(* Logix 5000 AddOnInstructionDefinition export AMP_Tuning_Params_StepSERVO; software revision 20.04 *)

ADD_ON_INSTRUCTION AMP_Tuning_Params_StepSERVO   (* revision 1.0 *)
// Applied Motion - Tuning Parameters StepSERVO AOI
// Help:
// The Tuning Parameters for StepSERVO AOI accepts all the required parameters for SCL commands VP, VI, KK, KC, KP, KD and KE, and then scales and issues these to the drive, one at a time.
VAR_IN_OUT
   MSG_Write : SINT[8]; {required}   // Message Write data tag
        [0]   // Message Reserved = 0
        [1]   // Message Type (16#01 or 16#02)
        [2]   // Type 1: Register Type 2: Opcode
        [3]   // Type 1: Opcode Type 2: Operand
        [4]   // Type 1: Parameter 1 Type 2: data MSB
        [5]   // Type 1: Parameter 2 Type 2: data LSB
        [6]   // Type 1: Parameter 3 Type 2: not used
        [7]   // Type 1: Parameter 4 Type 2: not used
   SendMsg : MESSAGE; {required}   // Message tag
   MSG_Response : SINT[8]; {required}   // Message Response data tag
        [0]   // Command Word
        [1]   // Jog Speed (0.25 rev/min)
        [2]   // Jog Acceleration (10 rev/s/s)
        [3]   // Jog Deceleration (10 rev/s/s)
        [4]   // Point-to-Point Velocity (0.25 rev/min)
        [5]   // Point-to-Point Acceleration (10 rev/s/s)
        [6]   // Point-to-Point Deceleration (10 rev/s/s)
        [7]   // Point-to-Point Distance (Motor steps)
        [9]   // (2x ASCII Letters in 16 lower word)
        [10]   // Data/Register 1
        [11]   // Data/Register 2
END_VAR
VAR_INPUT
   Configure : BOOL; {required}   // Start the Configuration
   VP : INT; {required}   // Velocity Mode Proportional Constant
   VI : INT; {required}   // Velocity Integrator Constant
   KP : INT; {required}   // Proportional Global Gain Value
   KK : INT; {required}   // Inertia Feedforward Gain
   KE : INT; {required}   // Differential Filter Gain Value
   KD : INT; {required}   // Damping Gain Value
   KC : INT; {required}   // Overall Servo Filter value
END_VAR
VAR_OUTPUT
   Sent : BOOL; {access Read Only, visible}   // All parameter settings have been sent to drive
   In_Progress : BOOL; {access Read Only, visible}   // The setting of parameters is in progress
   Done : BOOL; {access Read Only, visible}   // Parameters set without errors
   Error : BOOL; {access Read Only, visible}   // Configuration failed to complete - drive not ready or faulted
   State : DINT := 34; {access Read Only}   // Internal state of progress
END_VAR
VAR
   Loc_Start_ONS : BOOL; {access None}
   MSG_Active : BOOL;
END_VAR

ROUTINE Logic   (* ladder *)
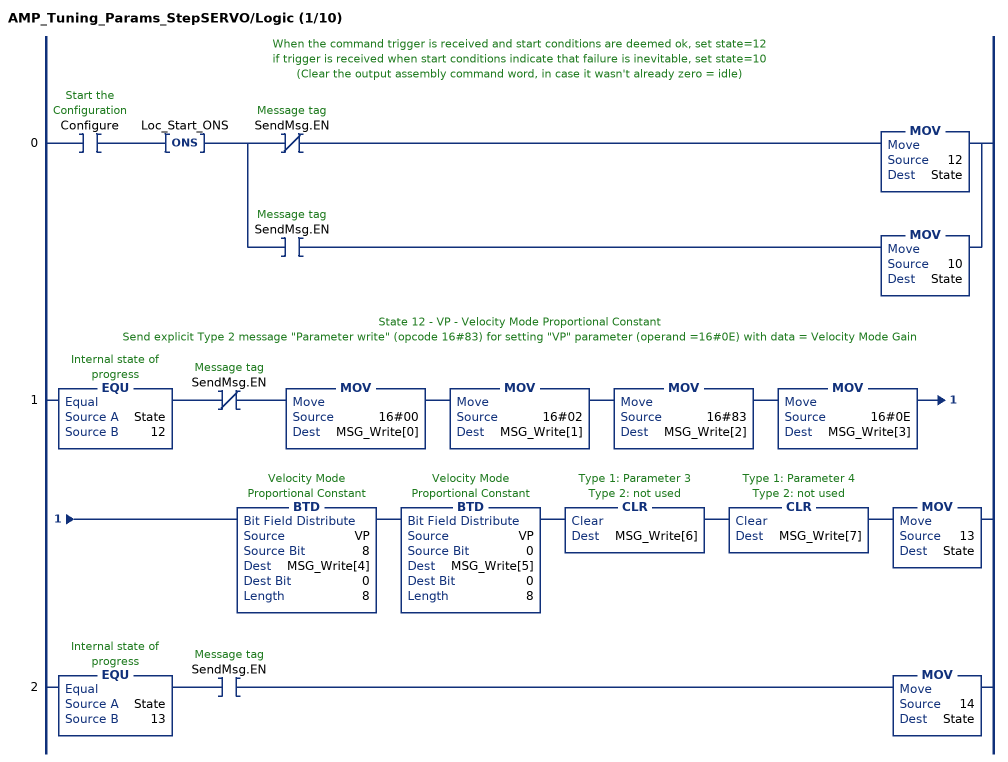
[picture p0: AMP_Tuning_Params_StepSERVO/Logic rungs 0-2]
   // When the command trigger is received and start conditions are deemed ok, set state=12
   // if trigger is received when start conditions indicate that failure is inevitable, set state=10
   // (Clear the output assembly command word, in case it wasn't already zero = idle)
   0: XIC(Configure)ONS(Loc_Start_ONS)[XIO(SendMsg.EN) MOV(12,State) ,XIC(SendMsg.EN) MOV(10,State) ];
   // State 12 - VP - Velocity Mode Proportional Constant
   // Send explicit Type 2 message "Parameter write" (opcode 16#83) for setting "VP" parameter (operand =16#0E) with data = Velocity Mode Gain
   1: EQU(State,12)XIO(SendMsg.EN)MOV(16#00,MSG_Write[0])MOV(16#02,MSG_Write[1])MOV(16#83,MSG_Write[2])MOV(16#0E,MSG_Write[3])BTD(VP,8,MSG_Write[4],0,8)BTD(VP,0,MSG_Write[5],0,8)CLR(MSG_Write[6])CLR(MSG_Write[7])MOV(13,State);
   2: EQU(State,13)XIC(SendMsg.EN)MOV(14,State);
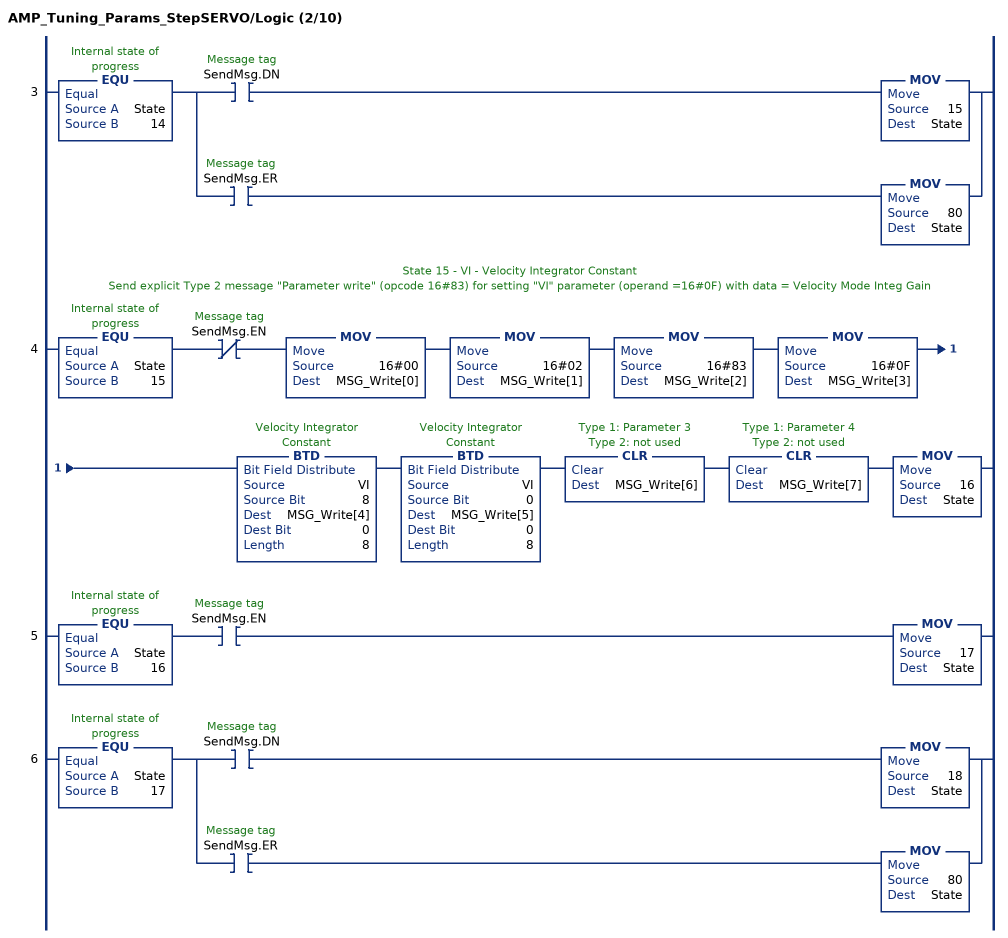
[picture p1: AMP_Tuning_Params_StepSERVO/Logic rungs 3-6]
   3: EQU(State,14)[XIC(SendMsg.DN) MOV(15,State) ,XIC(SendMsg.ER) MOV(80,State) ];
   // State 15 - VI - Velocity Integrator Constant
   // Send explicit Type 2 message "Parameter write" (opcode 16#83) for setting "VI" parameter (operand =16#0F) with data = Velocity Mode Integ Gain
   4: EQU(State,15)XIO(SendMsg.EN)MOV(16#00,MSG_Write[0])MOV(16#02,MSG_Write[1])MOV(16#83,MSG_Write[2])MOV(16#0F,MSG_Write[3])BTD(VI,8,MSG_Write[4],0,8)BTD(VI,0,MSG_Write[5],0,8)CLR(MSG_Write[6])CLR(MSG_Write[7])MOV(16,State);
   5: EQU(State,16)XIC(SendMsg.EN)MOV(17,State);
   6: EQU(State,17)[XIC(SendMsg.DN) MOV(18,State) ,XIC(SendMsg.ER) MOV(80,State) ];
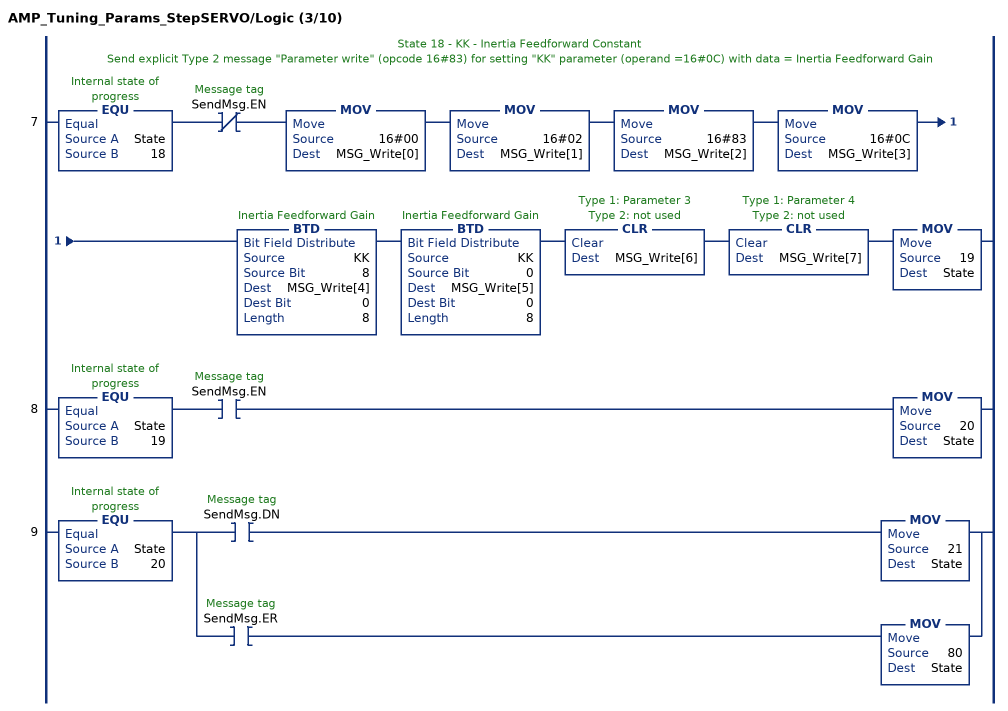
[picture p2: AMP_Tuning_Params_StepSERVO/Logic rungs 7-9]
   // State 18 - KK - Inertia Feedforward Constant
   // Send explicit Type 2 message "Parameter write" (opcode 16#83) for setting "KK" parameter (operand =16#0C) with data = Inertia Feedforward Gain
   7: EQU(State,18)XIO(SendMsg.EN)MOV(16#00,MSG_Write[0])MOV(16#02,MSG_Write[1])MOV(16#83,MSG_Write[2])MOV(16#0C,MSG_Write[3])BTD(KK,8,MSG_Write[4],0,8)BTD(KK,0,MSG_Write[5],0,8)CLR(MSG_Write[6])CLR(MSG_Write[7])MOV(19,State);
   8: EQU(State,19)XIC(SendMsg.EN)MOV(20,State);
   9: EQU(State,20)[XIC(SendMsg.DN) MOV(21,State) ,XIC(SendMsg.ER) MOV(80,State) ];
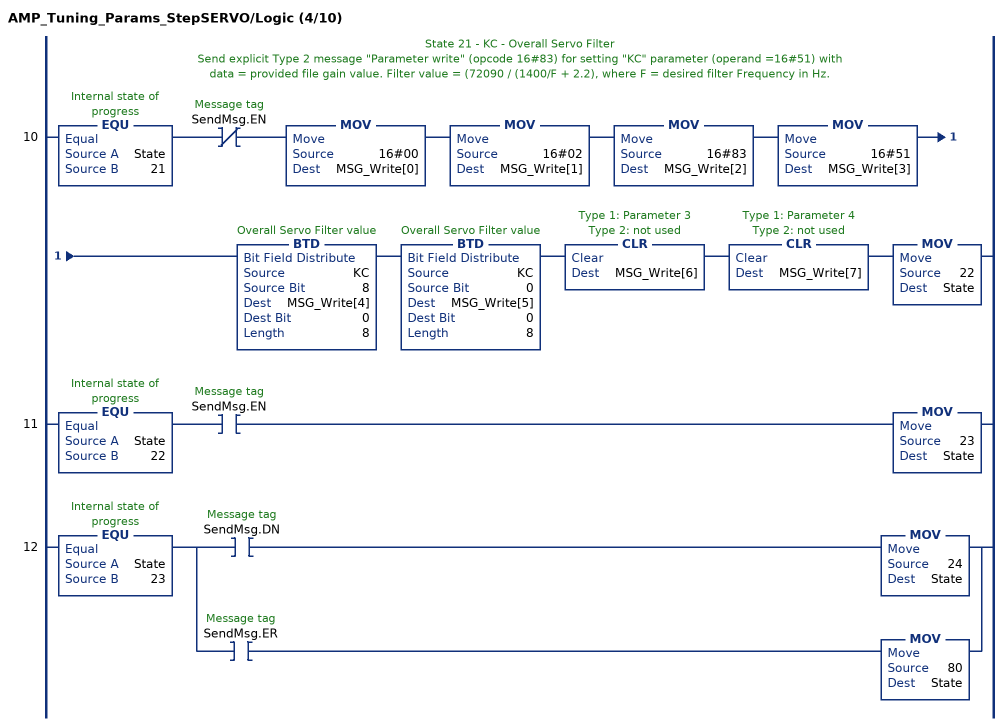
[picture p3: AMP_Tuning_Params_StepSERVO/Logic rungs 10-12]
   // State 21 - KC - Overall Servo Filter
   // Send explicit Type 2 message "Parameter write" (opcode 16#83) for setting "KC" parameter (operand =16#51) with
   // data = provided file gain value. Filter value = (72090 / (1400/F + 2.2), where F = desired filter Frequency in Hz.
   10: EQU(State,21)XIO(SendMsg.EN)MOV(16#00,MSG_Write[0])MOV(16#02,MSG_Write[1])MOV(16#83,MSG_Write[2])MOV(16#51,MSG_Write[3])BTD(KC,8,MSG_Write[4],0,8)BTD(KC,0,MSG_Write[5],0,8)CLR(MSG_Write[6])CLR(MSG_Write[7])MOV(22,State);
   11: EQU(State,22)XIC(SendMsg.EN)MOV(23,State);
   12: EQU(State,23)[XIC(SendMsg.DN) MOV(24,State) ,XIC(SendMsg.ER) MOV(80,State) ];
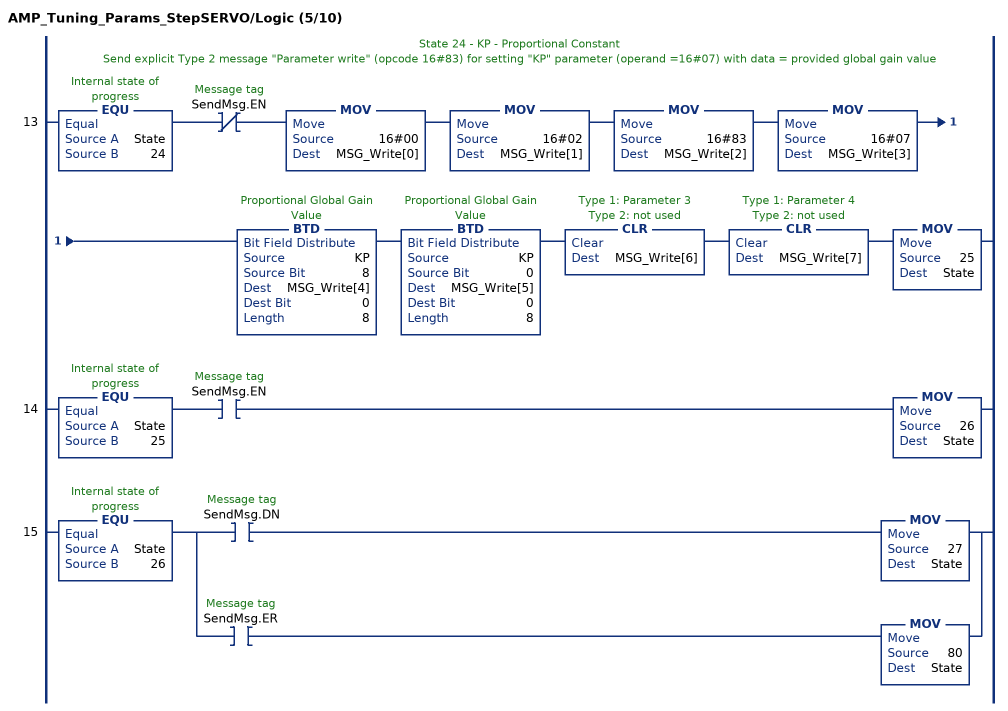
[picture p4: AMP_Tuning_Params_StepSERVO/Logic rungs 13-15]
   // State 24 - KP - Proportional Constant
   // Send explicit Type 2 message "Parameter write" (opcode 16#83) for setting "KP" parameter (operand =16#07) with data = provided global gain value
   13: EQU(State,24)XIO(SendMsg.EN)MOV(16#00,MSG_Write[0])MOV(16#02,MSG_Write[1])MOV(16#83,MSG_Write[2])MOV(16#07,MSG_Write[3])BTD(KP,8,MSG_Write[4],0,8)BTD(KP,0,MSG_Write[5],0,8)CLR(MSG_Write[6])CLR(MSG_Write[7])MOV(25,State);
   14: EQU(State,25)XIC(SendMsg.EN)MOV(26,State);
   15: EQU(State,26)[XIC(SendMsg.DN) MOV(27,State) ,XIC(SendMsg.ER) MOV(80,State) ];
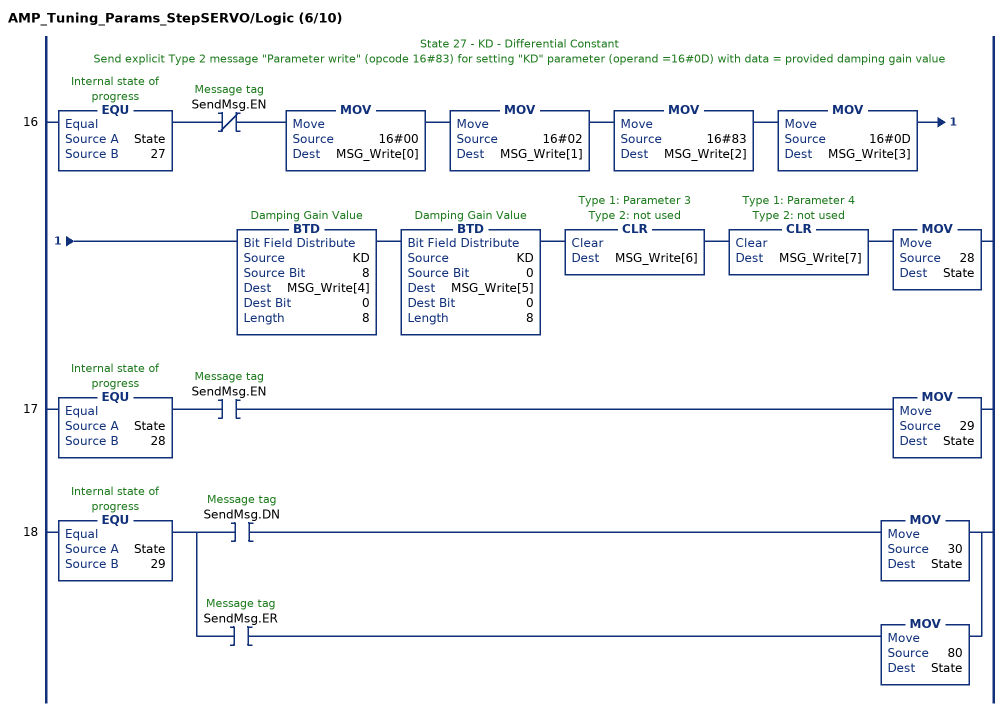
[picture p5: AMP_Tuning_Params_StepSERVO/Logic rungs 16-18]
   // State 27 - KD - Differential Constant
   // Send explicit Type 2 message "Parameter write" (opcode 16#83) for setting "KD" parameter (operand =16#0D) with data = provided damping gain value
   16: EQU(State,27)XIO(SendMsg.EN)MOV(16#00,MSG_Write[0])MOV(16#02,MSG_Write[1])MOV(16#83,MSG_Write[2])MOV(16#0D,MSG_Write[3])BTD(KD,8,MSG_Write[4],0,8)BTD(KD,0,MSG_Write[5],0,8)CLR(MSG_Write[6])CLR(MSG_Write[7])MOV(28,State);
   17: EQU(State,28)XIC(SendMsg.EN)MOV(29,State);
   18: EQU(State,29)[XIC(SendMsg.DN) MOV(30,State) ,XIC(SendMsg.ER) MOV(80,State) ];
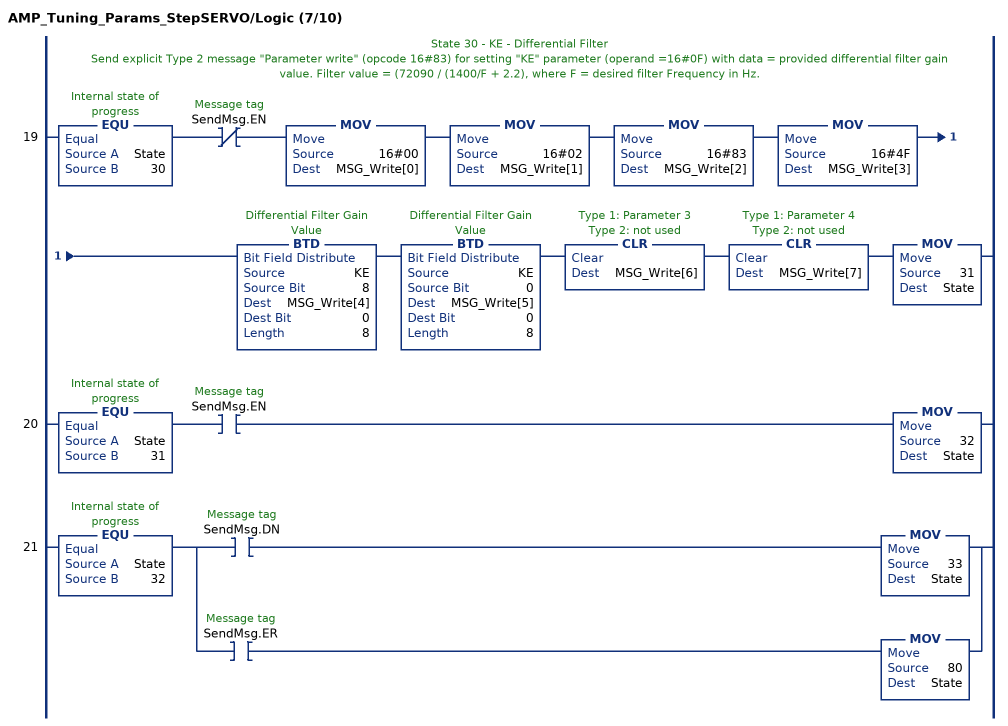
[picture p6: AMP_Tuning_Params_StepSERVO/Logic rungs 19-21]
   // State 30 - KE - Differential Filter
   // Send explicit Type 2 message "Parameter write" (opcode 16#83) for setting "KE" parameter (operand =16#0F) with data = provided differential filter gain value. Filter value = (72090 / (1400/F + 2.2), where F = desired filter Frequency in Hz.
   19: EQU(State,30)XIO(SendMsg.EN)MOV(16#00,MSG_Write[0])MOV(16#02,MSG_Write[1])MOV(16#83,MSG_Write[2])MOV(16#4F,MSG_Write[3])BTD(KE,8,MSG_Write[4],0,8)BTD(KE,0,MSG_Write[5],0,8)CLR(MSG_Write[6])CLR(MSG_Write[7])MOV(31,State);
   20: EQU(State,31)XIC(SendMsg.EN)MOV(32,State);
   21: EQU(State,32)[XIC(SendMsg.DN) MOV(33,State) ,XIC(SendMsg.ER) MOV(80,State) ];
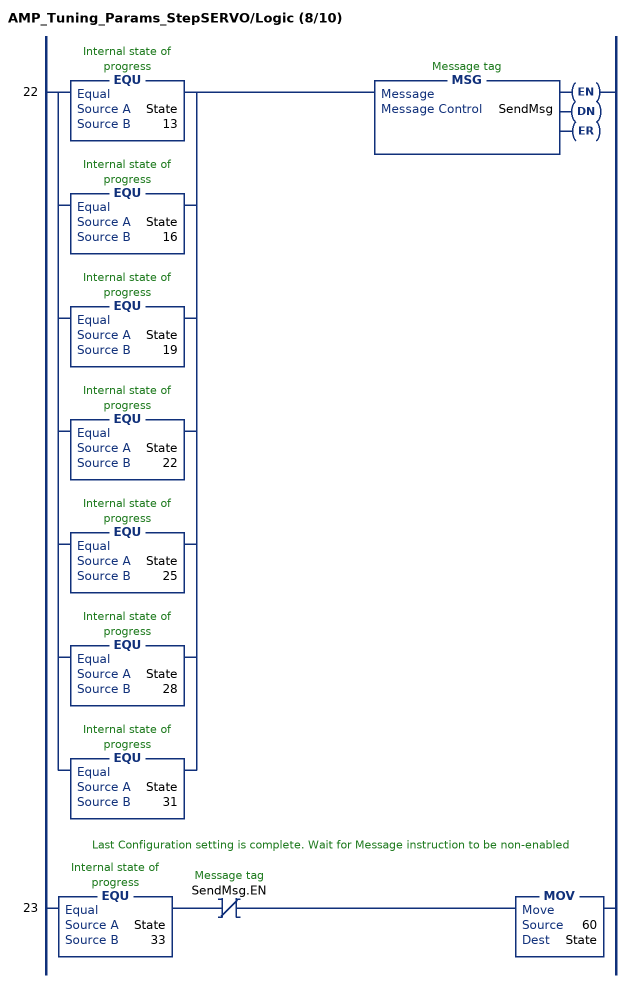
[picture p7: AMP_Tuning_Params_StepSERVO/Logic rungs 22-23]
   22: [EQU(State,13) ,EQU(State,16) ,EQU(State,19) ,EQU(State,22) ,EQU(State,25) ,EQU(State,28) ,EQU(State,31) ]MSG(SendMsg);
   // Last Configuration setting is complete. Wait for Message instruction to be non-enabled
   23: EQU(State,33)XIO(SendMsg.EN)MOV(60,State);
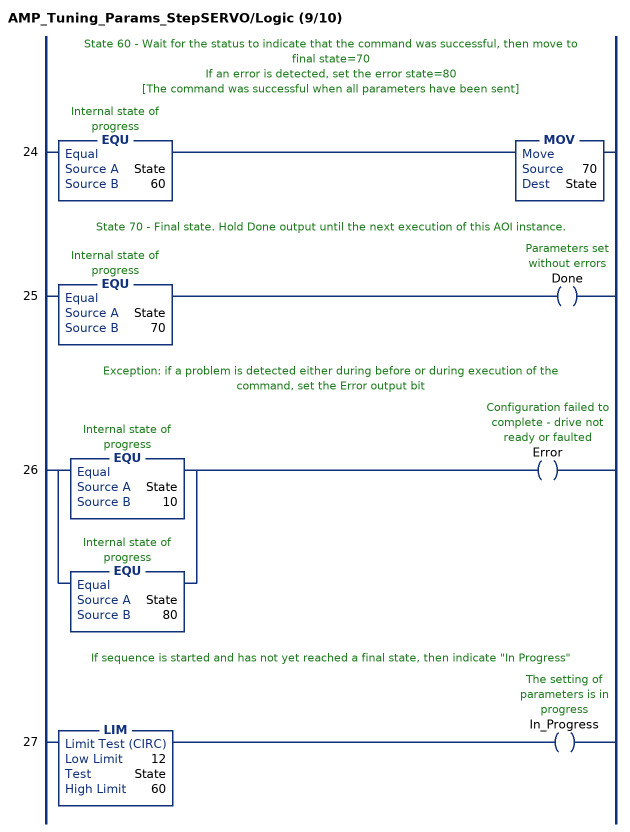
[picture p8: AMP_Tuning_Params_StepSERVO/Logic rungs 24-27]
   // State 60 - Wait for the status to indicate that the command was successful, then move to final state=70
   // If an error is detected, set the error state=80
   // [The command was successful when all parameters have been sent]
   24: EQU(State,60)MOV(70,State);
   // State 70 - Final state. Hold Done output until the next execution of this AOI instance.
   25: EQU(State,70)OTE(Done);
   // Exception: if a problem is detected either during before or during execution of the command, set the Error output bit
   26: [EQU(State,10) ,EQU(State,80) ]OTE(Error);
   // If sequence is started and has not yet reached a final state, then indicate "In Progress"
   27: LIM(12,State,60)OTE(In_Progress);
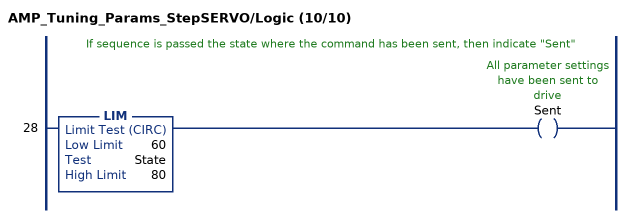
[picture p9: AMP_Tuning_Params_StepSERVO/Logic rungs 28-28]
   // If sequence is passed the state where the command has been sent, then indicate "Sent"
   28: LIM(60,State,80)OTE(Sent);
END_ROUTINE
END_ADD_ON_INSTRUCTION
